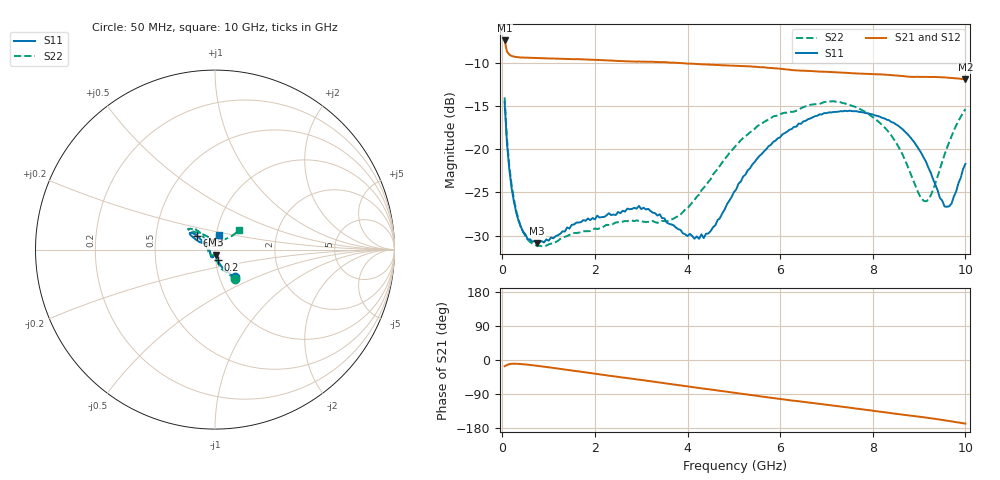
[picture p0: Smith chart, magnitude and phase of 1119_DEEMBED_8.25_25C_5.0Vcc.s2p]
!Hittite Microwave Corp.
!Digital Attenuator/PhaseShifter Rev 1.4.0
!Filename: C:\DATA\DATA\1119_DEEMBED_8.25_25C_5.0Vcc.s2p
!VNA ID: Agilent Technologies,N5224A,MY51441122,A.10.45.03
!Device type:
!2 Port Calibration.
!Temp(C): 25
!Lot Number:
!Serial Number:
!Operator:
!Misc:
!Attenuator:  8.250
# GHZ S DB R 50.0
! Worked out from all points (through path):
!   200 points, 50 MHz to 10 GHz, reference 50 ohm
!   highest |S21| = -7.40 dB at 50 MHz (marker M1); lowest = -11.9 dB at 10 GHz (marker M2)
!   group delay of S21, straight-line fit = 45.1 ps
!   lowest |S11| = -30.9 dB at 750 MHz (marker M3), VSWR 1.06, Z = 50.3 - j2.86 ohm
!   |S11| at or under -10 dB: start of sweep to end of sweep
!   |S22| runs from -31.2 to -14.0 dB; largest |S21 - S12| = 0.00078
!   S11 on the Smith chart (normalised r, x): 50 MHz: 1.18, -0.37; 200 MHz: 1.02, -0.12; 6.15 GHz: 0.81, +0.13; 10 GHz: 1.03, +0.16
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0.05  -14.53 -54.1  -7.40 -16.5  -7.40 -16.5  -14.00 -55.4
0.1  -19.22 -67.9  -8.66 -13.2  -8.65 -13.2  -18.72 -70.8
0.2  -24.46 -75.0  -9.19 -10.2  -9.19 -10.2  -24.11 -80.8
0.4  -28.97 -77.7  -9.37 -10.6  -9.37 -10.6  -28.98 -86.4
0.75  -30.86 -83.2  -9.44 -15.3  -9.44 -15.3  -31.16 -92.3
1.75  -28.20 -103.5  -9.59 -31.8  -9.59 -31.8  -29.50 -108.4
2.95  -26.56 -113.4  -9.84 -51.8  -9.85 -51.8  -28.30 -146.1
3.4  -27.52 -124.2  -9.90 -59.5  -9.91 -59.5  -28.39 -166.4
3.85  -29.35 -139.8  -10.02 -67.2  -10.03 -67.3  -27.55 169.5
4.35  -30.28 -169.8  -10.17 -75.4  -10.18 -75.5  -24.45 145.2
5.05  -24.67 152.5  -10.33 -87.0  -10.34 -87.0  -19.55 131.4
5.55  -20.78 144.7  -10.49 -95.5  -10.51 -95.5  -17.17 132.1
6.15  -17.97 142.7  -10.76 -105.3  -10.78 -105.3  -15.76 134.5
6.7  -16.30 143.6  -10.95 -113.5  -10.95 -113.4  -14.81 139.9
7.65  -15.60 148.0  -11.22 -128.2  -11.21 -128.2  -15.14 142.9
8.35  -16.64 150.1  -11.39 -139.6  -11.38 -139.6  -18.04 132.7
8.75  -18.24 152.3  -11.59 -146.0  -11.58 -145.9  -21.92 118.6
8.999999  -20.03 153.8  -11.62 -149.5  -11.62 -149.6  -25.25 100.8
9.15  -21.44 153.3  -11.62 -151.9  -11.63 -151.9  -26.03 81.8
9.6  -26.66 116.6  -11.70 -160.1  -11.71 -160.1  -19.87 41.2
9.7  -26.30 100.3  -11.74 -161.9  -11.75 -162.0  -18.49 38.9
10  -21.70 74.4  -11.91 -167.8  -11.92 -167.8  -15.35 38.8
